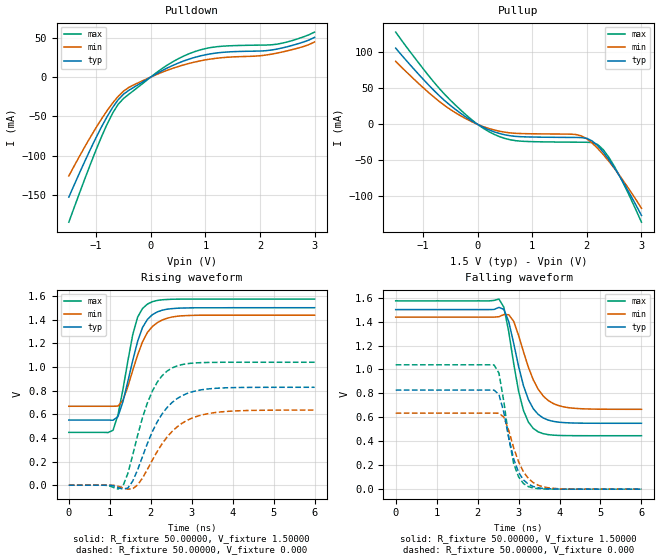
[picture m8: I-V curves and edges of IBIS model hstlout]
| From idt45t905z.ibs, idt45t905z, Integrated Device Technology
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|   Model hstlout
[Model]   hstlout
Model_type   Output
Polarity   Non-Inverting
Vmeas =  0.75000V
C_comp   5.00000pF   5.00000pF   5.00000pF
[Temperature Range]   45.00000   0.14000k   -30.00000
[Voltage Range]   1.50000V   1.40000V   1.60000V
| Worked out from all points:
|   slope of the pulldown table from 0 to 0.225 V, typ, clamps not added: 25.7 ohm
|   slope of the pullup table from 0 to 0.225 V, typ, clamps not added: 27.7 ohm
|   rising waveform, R_fixture 50.00000, V_fixture 1.50000: 20-80 % time 431ps typ, 479ps min, 378ps max; typ from 0.55 V to 1.5 V
|   rising waveform, R_fixture 50.00000, V_fixture 0.000: 20-80 % time 697ps typ, 796ps min, 572ps max; typ from 0 V to 0.828 V
|   falling waveform, R_fixture 50.00000, V_fixture 1.50000: 20-80 % time 433ps typ, 506ps min, 368ps max; typ from 1.5 V to 0.55 V
|   falling waveform, R_fixture 50.00000, V_fixture 0.000: 20-80 % time 350ps typ, 417ps min, 296ps max; typ from 0.828 V to 0 V
[Pulldown]
| voltage   I(typ)   I(min)   I(max)
-1.5V     -152.2mA   -125.4mA   -184mA
-1V       -76.61mA   -64mA      -92.15mA
-700mV    -38.83mA   -33.15mA   -46.03mA
-600mV    -29.09mA   -24.77mA   -34.85mA
-400mV    -16.8mA    -13.12mA   -21.77mA
100mV     4.071mA    3.04mA     5.393mA
500mV     17.6mA     13.29mA    23.07mA
900mV     26.67mA    20.45mA    34.32mA
1.3V      31.24mA    24.53mA    39.05mA
2.3V      35.32mA    30.19mA    41.59mA
2.7V      42.32mA    36.77mA    48.64mA
3V        50.37mA    44.55mA    57.01mA
[Pullup]
| voltage   I(typ)   I(min)   I(max)
-1.5V     106mA      87.68mA    128.3mA
-1V       63.03mA    51.23mA    77.62mA
-600mV    32.8mA     26mA       41.46mA
-100mV    4.501mA    3.42mA     5.936mA
200mV     -7.39mA    -5.559mA   -9.876mA
700mV     -16.74mA   -12.49mA   -22.72mA
1.8V      -18.22mA   -14.08mA   -24.77mA
2V        -19.46mA   -20.18mA   -24.89mA
2.2V      -29.78mA   -33.53mA   -28.11mA
2.3V      -38.45mA   -41.87mA   -35.18mA
2.5V      -59.91mA   -60.81mA   -57.87mA
3V        -126.6mA   -116.6mA   -136mA
[Ramp]
| variable   typ   min   max
dV/dt_r   0.49656/0.71193n   0.38106/0.80841n   0.62340/0.57907n
dV/dt_f   0.56976/0.43601n   0.47046/0.50463n   0.67134/0.37568n
R_load = 50.00000
[Rising Waveform]
R_fixture = 50.00000
V_fixture = 1.50000
C_fixture = 0.000F
R_dut = 2.40000m
L_dut = 0.90000nH
C_dut = 60.00000fF
| time   V(typ)   V(min)   V(max)
0s        550.4mV    667.1mV    446.5mV
1.08ns    549mV      667mV      464.2mV
1.2ns     579.7mV    669mV      595.6mV
1.32ns    704mV      716.8mV    806.3mV
1.56ns    1.053V     969.5mV    1.272V
1.68ns    1.216V     1.101V     1.421V
1.92ns    1.401V     1.292V     1.53V
2.16ns    1.464V     1.374V     1.562V
2.64ns    1.496V     1.427V     1.572V
6ns       1.5V       1.437V     1.573V
[Rising Waveform]
R_fixture = 50.00000
V_fixture = 0.000
C_fixture = 0.000F
R_dut = 2.40000m
L_dut = 0.90000nH
C_dut = 60.00000fF
| time   V(typ)   V(min)   V(max)
0s        0V         0V         0V
1.32ns    -33.27mV   -22.6mV    -8.722mV
1.44ns    -24.62mV   -33.46mV   98.83mV
1.56ns    34.44mV    -30.36mV   254.6mV
1.92ns    354.3mV    134.5mV    696.6mV
2.16ns    536.2mV    286mV      871.2mV
2.52ns    698.7mV    454.1mV    991mV
2.88ns    774.2mV    546.7mV    1.026V
3.48ns    816.2mV    609.7mV    1.038V
6ns       827.5mV    635.1mV    1.039V
[Falling Waveform]
R_fixture = 50.00000
V_fixture = 1.50000
C_fixture = 0.000F
R_dut = 2.40000m
L_dut = 0.90000nH
C_dut = 60.00000fF
| time   V(typ)   V(min)   V(max)
0s        1.5V       1.437V     1.573V
2.52ns    1.518V     1.44V      1.588V
2.64ns    1.502V     1.458V     1.521V
2.76ns    1.399V     1.457V     1.315V
2.88ns    1.219V     1.402V     1.05V
3.12ns    863.8mV    1.147V     656.6mV
3.36ns    671.7mV    912.5mV    507.1mV
3.6ns     595.1mV    778.9mV    463.7mV
3.96ns    560.5mV    699.8mV    449.1mV
6ns       550.4mV    667.1mV    446.5mV
[Falling Waveform]
R_fixture = 50.00000
V_fixture = 0.000
C_fixture = 0.000F
R_dut = 2.40000m
L_dut = 0.90000nH
C_dut = 60.00000fF
| time   V(typ)   V(min)   V(max)
0s        827.6mV    635.2mV    1.039V
2.4ns     827.6mV    635.2mV    1.038V
2.52ns    792mV      634.7mV    969.9mV
2.64ns    641.5mV    602.1mV    733.1mV
2.76ns    427.6mV    490.8mV    431.4mV
2.88ns    253mV      345.8mV    214mV
3ns       141.1mV    228.4mV    102.9mV
3.24ns    41.33mV    89.23mV    20.98mV
3.84ns    1.877mV    7.2mV      492.1uV
6ns       948.2nV    3.386uV    2.24uV
